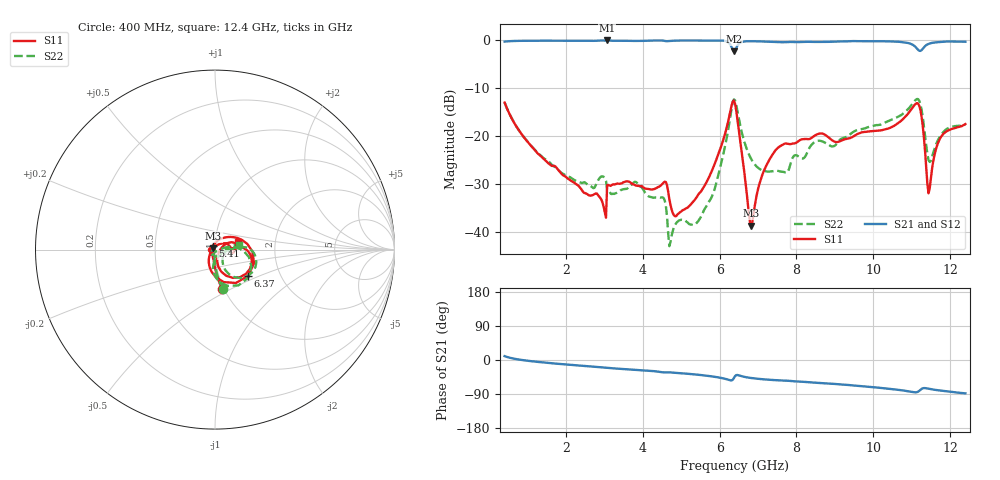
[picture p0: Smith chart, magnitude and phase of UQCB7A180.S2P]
!  Part Number  UQCB7A180	Mounting Orientation: Vertical
!  Description: RF capacitors
!  Application: Coupling, Bypass, Tuning, DC Block
!  Filters, Matching
# GHZ S DB R 50
! Freq  |S11|  S11 Ph  |S21|  S21 Ph  |S12|  S12 Ph  |S22|  S22 Ph
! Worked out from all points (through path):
!   401 points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, 400 MHz to 12.4 GHz, reference 50 ohm
!   highest |S21| = 0.00 dB at 3.07 GHz (marker M1); lowest = -2.3 dB at 6.37 GHz (marker M2)
!   group delay of S21, straight-line fit = 20.8 ps
!   lowest |S11| = -38.7 dB at 6.82 GHz (marker M3), VSWR 1.02, Z = 49.1 + j0.757 ohm
!   |S11| at or under -10 dB: start of sweep to end of sweep
!   |S22| runs from -42.9 to -12.2 dB; largest |S21 - S12| = 0.0016
!   S11 on the Smith chart (normalised r, x): 400 MHz: 0.98, -0.46; 5.41 GHz: 0.97, +0.04; 6.37 GHz: 1.38, -0.43; 12.4 GHz: 1.29, +0.11
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0.4  -12.96 -79.6  -0.24 10.2  -0.25 10.2  -12.95 -79.0
1.24  -23.33 -95.6  -0.06 -4.8  -0.07 -4.8  -23.24 -90.9
2.41  -31.17 -126.5  -0.06 -15.3  -0.06 -15.2  -29.73 -85.5
3.07  -30.18 -103.9  0.00 -20.8  -0.01 -20.8  -31.08 -108.9
4.42  -30.51 -153.8  -0.01 -31.1  -0.01 -31.1  -32.78 -138.1
4.57  -29.46 -173.3  -0.10 -32.7  -0.11 -32.7  -33.39 -155.1
4.72  -34.28 158.6  -0.08 -32.8  -0.09 -32.8  -42.05 -119.5
4.87  -36.63 173.4  -0.03 -33.9  -0.04 -33.9  -38.09 -99.5
5.41  -32.61 124.8  -0.01 -38.6  -0.01 -38.6  -37.99 -52.2
5.86  -26.01 74.9  -0.01 -44.2  -0.01 -44.1  -31.25 -0.7
6.22  -16.95 26.9  -0.40 -51.9  -0.41 -51.9  -18.76 6.1
6.37  -12.54 -38.3  -2.30 -47.8  -2.31 -47.8  -12.30 -40.4
6.4  -13.18 -58.0  -2.13 -42.7  -2.14 -42.6  -12.46 -56.7
6.82  -38.66 138.7  -0.16 -47.5  -0.16 -47.5  -24.69 -88.9
7.09  -28.54 52.8  -0.21 -50.5  -0.21 -50.5  -27.03 -69.0
7.42  -23.29 30.5  -0.33 -53.0  -0.33 -53.0  -27.20 -47.5
8.41  -20.23 2.4  -0.30 -59.4  -0.30 -59.4  -21.62 -6.1
10.42  -18.28 4.1  -0.20 -76.1  -0.20 -76.1  -16.72 5.6
11.17  -13.19 -37.9  -1.97 -83.5  -1.97 -83.5  -12.25 -30.4
11.47  -30.89 -1.8  -0.63 -76.3  -0.63 -76.4  -25.34 -23.3
11.77  -20.06 24.4  -0.30 -80.9  -0.30 -80.9  -19.64 13.6
12.4  -17.44 18.0  -0.27 -88.0  -0.28 -88.1  -17.46 10.4
